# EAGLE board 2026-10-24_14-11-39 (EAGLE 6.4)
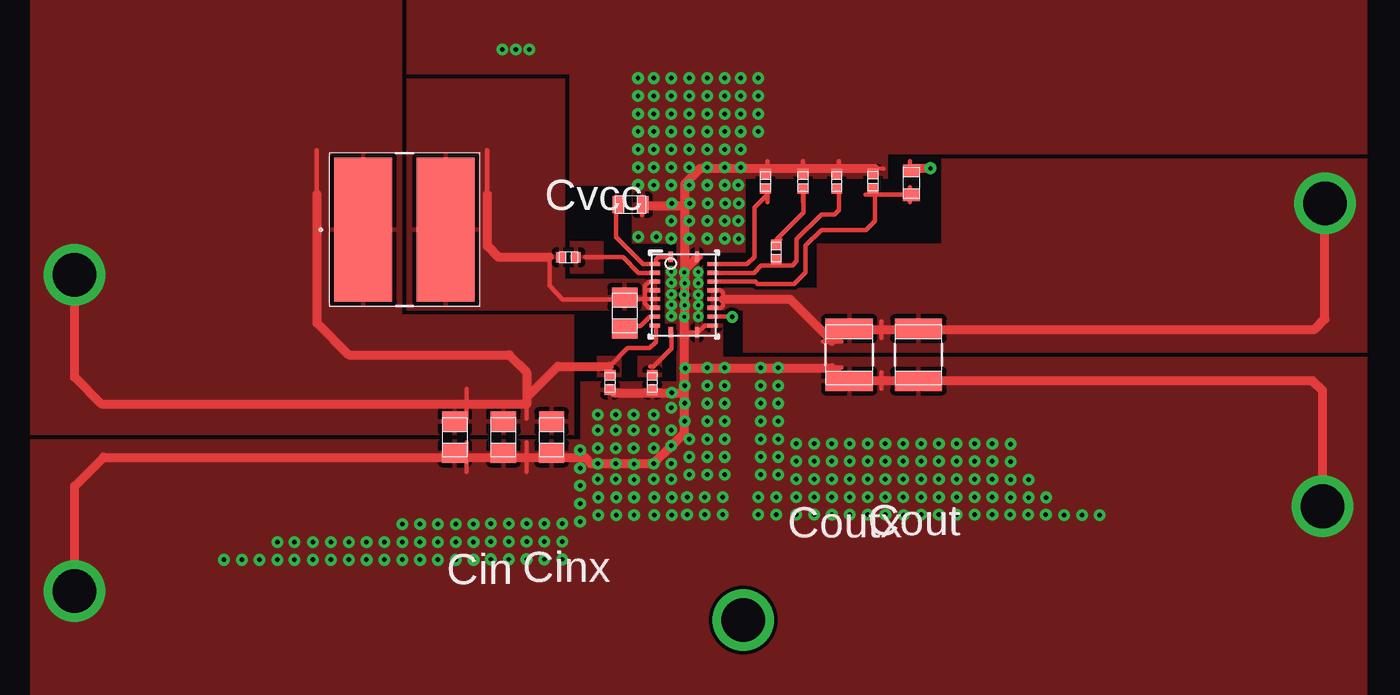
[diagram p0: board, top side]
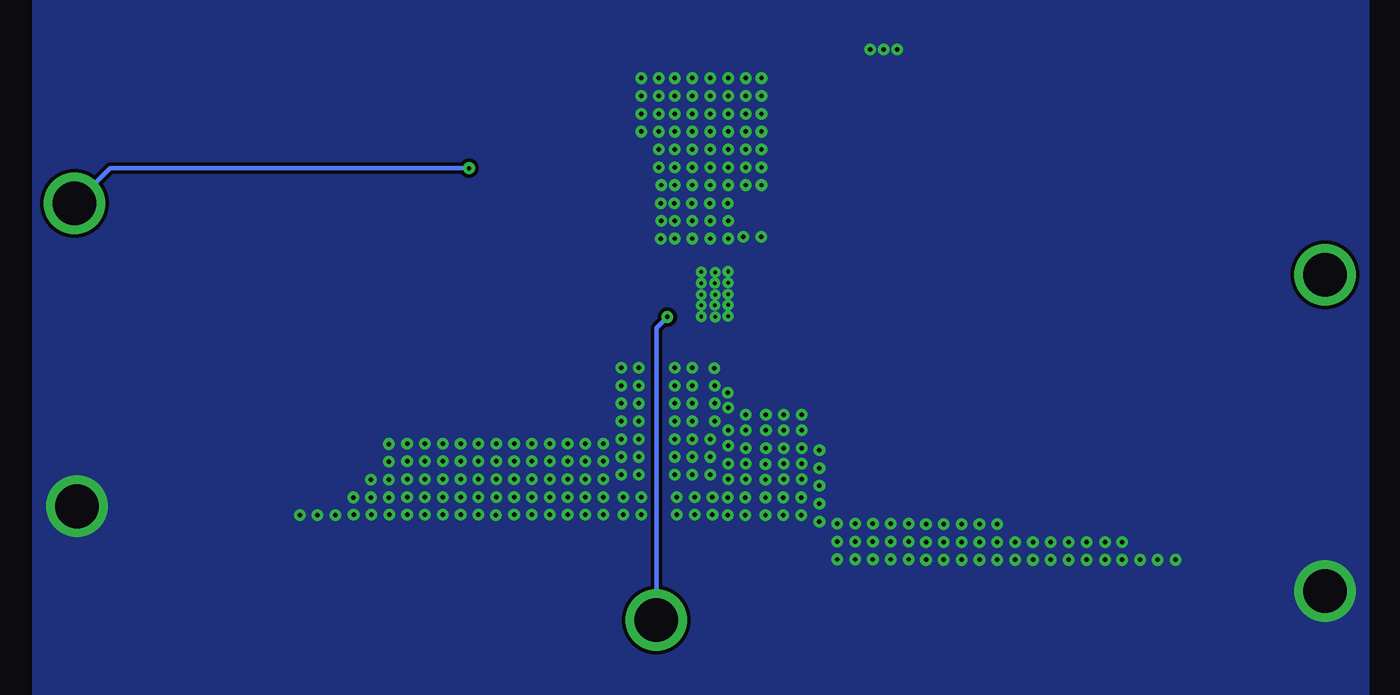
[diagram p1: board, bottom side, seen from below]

No outline drawn. Coordinates in mm, seen from the top.
Copper layers ((1*2)+(15*16)): TOP / INTERNAL1 / layer 15 / BOTTOM

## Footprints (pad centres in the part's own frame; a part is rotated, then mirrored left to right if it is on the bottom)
0805 = smd 1.118 x 1.448: 1 -0.902,0; 2 0.902,0
0402 = smd 0.559 x 0.61: 1 -0.419,0; 2 0.419,0
1210_280 = smd 1.118 x 2.692: 1 -1.499,0; 2 1.499,0
0603 = smd 0.66 x 0.965: 1 -0.699,0; 2 0.699,0
TP-1502 = drill 0.813 pad 1.651 round: 1 0,0
VLP8040 = smd 3.302 x 8.204: 1 -2.349,0; 2 2.349,0
RHL0020A = smd 0.24 x 0.6: 1 -0.75,2.15; 10 -0.75,-2.15; 11 0.75,-2.15; 20 0.75,2.15 | smd 0.6 x 0.24: 2 -1.65,1.75; 3 -1.65,1.25; 4 -1.65,0.75; 5 -1.65,0.25; 6 -1.65,-0.25; 7 -1.65,-0.75; 8 -1.65,-1.25; 9 -1.65,-1.75; 12 1.65,-1.75; 13 1.65,-1.25; 14 1.65,-0.75; 15 1.65,-0.25; 16 1.65,0.25; 17 1.65,0.75; 18 1.65,1.25; 19 1.65,1.75 | smd 0.3 x 0.3: 21 0,0

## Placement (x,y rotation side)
Cbst  [0805]  60.55,53.7 270 top
Ccomp  [0402]  70.71,61.19 90 top
Ccomp2  [0402]  72.64,61.19 90 top
Cin2  [0402]  59.72,49.73 270 top
Cin_1  [0805]  56.39,46.61 270 top
Cin_2  [0805]  53.64,46.61 270 top
Cin_3  [0805]  50.88,46.61 270 top
Cout_1  [1210_280]  73.36,51.31 270 top
Cout_2  [1210_280]  77.29,51.31 270 top
Css  [0402]  62.13,49.73 270 top
Cvcc_1  [0603]  60.88,59.87 0 top
Cvcc_2  [0603]  60.88,59.87 0 top
GND  [TP-1502]  29.18,37.85 270 top
GND1  [TP-1502]  100.28,42.65 270 top
L1  [VLP8040]  48.01,58.45 0 top
MODE  [TP-1502]  67.28,36.2 270 top
Rcomp  [0402]  69.19,57.18 90 top
Rfbb  [0402]  74.7,61.21 90 top
Rfbt  [0603]  76.89,61.11 270 top
Rlim  [0402]  68.58,61.19 90 top
Rt  [0402]  57.35,56.87 0 top
U1  [RHL0020A]  63.93,54.74 0 top
VIN  [TP-1502]  29.18,55.83 270 top
VOUT  [TP-1502]  100.38,59.89 270 top

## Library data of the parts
Cbst = ultra-librarian; RefDes: Cbst; Type: 08053C104KAT2A
Ccomp = ultra-librarian; RefDes: Ccomp; Type: GRM1555C1E751JA01D
Ccomp2 = ultra-librarian; RefDes: Ccomp2; Type: GRM1555C1E390JA01D
Cin2 = ultra-librarian; RefDes: Cin2; Type: GRM155R71A104KA01D
Cin_1-Cin_3 Cout_1 Cout_2 Cvcc_1 Cvcc_2 = ultra-librarian
Css = ultra-librarian; RefDes: Css; Type: GRM155R71C822KA01D
GND = ultra-librarian; RefDes: GND; Type: TP-1502
GND1 = ultra-librarian; RefDes: GND1; Type: TP-1502
L1 = ultra-librarian; RefDes: L1; Type: VLP8040T-1R0N
MODE = ultra-librarian; RefDes: MODE; Type: TP-1502
Rcomp = ultra-librarian; RefDes: Rcomp; Type: CRCW040226K7FKED
Rfbb = ultra-librarian; RefDes: Rfbb; Type: CRCW040269K8FKED
Rfbt = ultra-librarian; RefDes: Rfbt; Type: RC0603FR-07220KL
Rlim = ultra-librarian; RefDes: Rlim; Type: CRCW0402154KFKED
Rt = ultra-librarian; RefDes: Rt; Type: CRCW0402267KFKED
U1 = ultra-librarian; RefDes: U1; Type: TPS61088RHLR
VIN = ultra-librarian; RefDes: VIN; Type: TP-1502
VOUT = ultra-librarian; RefDes: VOUT; Type: TP-1502

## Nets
0: Ccomp2.2 Ccomp.2 Cin2.2 Cin_1.2 Cin_2.2 Cin_3.2 Cout_1.2 Cout_2.2 Css.2 Cvcc_1.2 Cvcc_2.2 GND1.1 GND.1 Rfbb.2 Rlim.2 U1.11 U1.12 U1.20 U1.21
2: Cin2.1 Cin_1.1 Cin_2.1 Cin_3.1 L1.1 U1.9 VIN.1
3: Ccomp.1 Rcomp.2
4: Cvcc_1.1 Cvcc_2.1 U1.1 U1.2
5: Ccomp2.1 Rcomp.1 U1.18
9: Cout_1.1 Cout_2.1 Rfbt.1 U1.14 U1.15 U1.16 VOUT.1
11: Rfbb.1 Rfbt.2 U1.17
12: Cbst.1 L1.2 Rt.1 U1.4 U1.5 U1.6 U1.7
14: Rlim.1 U1.19
17: Css.1 U1.10
18: Cbst.2 U1.8
19: Rt.2 U1.3
25: MODE.1 U1.13

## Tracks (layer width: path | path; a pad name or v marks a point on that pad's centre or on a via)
0  (via drill 0.2 pad 0.48, 0.25 pad 0.51, 2.49 pad 3.48)
  TOP 0.254: 65.61,52.98 65.13,52.98 64.72,52.58 63.98,52.58 63.96,52.58 | 74.27,61.94 75.31,61.94 | 72.76,61.52 72.76,62.36 | 70.73,61.52 70.73,62.36 | 68.69,61.52 68.69,62.36 | 71.86,50.58 72.9,50.58 | 61.56,59.28 61.56,60.33 | 54.97,44.63 54.97,46.3 | 75.18,49.38 75.18,50.32 | 51.54,44.63 51.54,46.3
  TOP 0.508: 63.98,59.82 63.98,60.98 63.98,61.06 64.87,61.95 68.71,61.95 70.74,61.95 | 63.98,59.82 63.98,58.95 63.98,56.16 | 63.98,56.16 v63.98,55.4 v63.98,54.13 63.98,53.49 v63.96,53.47 63.96,52.58 63.96,50.67 | 61.57,59.82 63.98,59.82 | 63.96,49.4 63.96,50.67 | 63.96,49.4 63.96,46.86 v63.22,46.13 v62.2,45.11 v60.05,45.11 v59.03,45.11 58.62,45.11 58.29,45.47 54.99,45.47 51.56,45.47 30.86,45.47 29.21,43.81 v29.21,37.85 | 59.69,49.4 59.94,49.15 62,49.15 63.73,49.15 63.96,49.4 | 63.96,50.67 64.03,50.57 v69.32,50.57 72.36,50.57 73.13,49.84 75.18,49.84 99.75,49.84 100.33,49.28 v100.33,42.67 | 63.98,56.16 64.72,56.9 | 59.69,49.4 | 63.96,49.4 | 70.74,61.95 72.77,61.95 74.8,61.95 | 70.74,61.95 | 74.8,61.95 | 61.57,59.82
  other vias: 63.22,54.76 63.96,56.01 64.74,54.74 63.22,53.52 63.22,54.15 63.22,56.06 37.72,39.62 39.75,39.62 41.73,39.62 67.06,59.94 87.63,42.16 86.61,42.16 85.6,42.16 84.58,43.18 83.57,43.18 82.55,45.21 82.55,44.2 82.55,43.18 82.55,46.23 40.77,39.62 40.77,40.64 41.73,40.64 42.8,39.62 42.8,40.64 43.81,39.62 43.81,40.64 44.83,39.62 44.83,40.64 45.85,39.62 45.85,40.64 55.12,68.71 76.45,42.16 64.01,50.55 69.19,43.21 58.01,44.86 63.22,48.29 73.38,46.25 63.96,54.74 48.9,40.64 48.9,39.62 48.9,41.66 60.07,42.16 60.07,43.18 47.88,41.66 47.88,39.62 47.88,40.64 46.86,40.64 46.86,39.62 61.09,43.18 61.09,42.16 49.91,41.66 49.91,39.62 49.91,40.64 50.93,40.64 50.93,39.62 50.93,41.66 62.23,42.16 62.23,43.18 64.74,54.13 64.74,53.49 64.74,55.4 63.22,55.42 64.74,56.03 68.3,50.57 66.27,50.57 65.25,50.57 68.3,49.56 65.25,49.56 66.27,49.56 66.27,47.52 63.22,47.02 63.98,47.52 65.25,47.52 60.05,47.9 59.03,47.9 68.17,43.21 66.14,43.21 58.01,45.87 64.11,43.21 63.25,43.18 65.13,43.21 69.32,49.56 64.11,42.19 63.25,42.16 69.19,42.19 65.13,42.19 66.14,42.19 68.17,42.19 61.06,47.02 59.03,47.02 60.05,47.02 62.2,47.02 79.48,45.24 74.4,45.24 72.36,45.24 73.38,45.24 78.46,45.24 75.41,45.24 76.43,45.24 77.44,45.24 70.33,45.24 69.32,47.52 68.3,47.52 71.35,45.24 71.35,44.22 68.3,46.51 69.32,46.51 70.33,44.22 77.44,44.22 76.43,44.22 75.41,44.22 78.46,44.22 73.38,44.22 72.36,44.22 74.4,44.22 79.48,44.22 60.05,46 59.03,46 58.01,43.84 61.06,46 55.98,41.68 54.97,41.68 53.95,41.68 57,41.68 51.94,41.66 52.93,41.68 65.25,46.51 64.24,46.51 66.27,46.51 66.27,44.48 63.22,44.22 64.24,44.48 65.25,44.48 52.93,39.65 51.94,39.62 57,39.65 53.95,39.65 54.97,39.65 55.98,39.65 61.09,44.2 58.01,41.81 59.03,44.22 60.05,44.22 62.2,44.22 79.48,42.19 74.4,42.19 72.36,42.19 73.38,42.19 78.46,42.19 75.41,42.19 77.44,42.19 70.33,42.19 69.32,44.48 68.3,44.48 71.35,42.19 71.35,43.21 68.3,45.49 69.32,45.49 70.33,43.21 77.44,43.21 76.43,43.21 75.41,43.21 78.46,43.21 73.38,43.21 72.36,43.21 74.4,43.21 79.48,43.21 58.01,42.82 55.98,40.67 54.97,40.67 53.95,40.67 57,40.67 51.94,40.64 52.93,40.67 65.25,45.49 64.24,45.49 63.22,45.11 66.27,45.49 83.54,42.19 80.49,42.19 81.51,42.19 82.52,42.19 84.56,42.19 65.25,57.94 63.22,57.94 64.24,57.94 66.27,57.94 65.25,58.95 63.22,58.95 64.24,58.95 66.27,58.95 66.29,59.94 63.25,59.94 64.26,59.94 65.28,59.94 66.27,60.99 63.22,60.99 64.24,60.99 65.25,60.99 67.03,60.99 61.32,62 67.16,62 65.25,62 64.24,62 63.22,62 66.27,62 62.2,63.02 66.27,63.02 63.22,63.02 64.24,63.02 65.25,63.02 67.16,63.02 68.17,64.03 67.16,64.03 65.25,64.03 64.24,64.03 63.22,64.03 66.27,64.03 62.2,64.03 62.2,65.05 66.27,65.05 63.22,65.05 64.24,65.05 65.25,65.05 67.16,65.05 68.17,65.05 68.17,66.07 67.16,66.07 65.25,66.07 64.24,66.07 63.22,66.07 66.27,66.07 62.2,66.07 68.17,67.08 67.16,67.08 65.25,67.08 64.24,67.08 63.22,67.08 66.27,67.08 62.2,67.08 61.32,60.99 62.2,62 62.2,60.99 71.35,46.25 68.3,48.54 69.32,48.54 70.33,46.25 77.44,46.25 76.43,46.25 75.41,46.25 78.46,46.25 72.36,46.25 74.4,46.25 79.48,46.25 62.2,47.9 61.06,47.9 65.25,48.54 66.27,48.54 81.51,46.25 80.49,46.25 81.51,43.21 80.49,43.21 81.51,44.22 80.49,44.22 80.49,45.24 81.51,45.24 61.32,67.08 61.32,66.07 61.32,65.05 61.32,64.03 61.32,63.02 63.25,49.15 59.05,42.16 59.05,43.18 53.59,68.71 38.73,39.62 54.36,68.71 63.98,49.56 63.98,48.54 62.2,46 61.09,45.09 83.57,44.2 62.36,58.04 61.34,58.04 67.06,57.91 67.03,58.95
  pour TOP: 58.04,49.78 63.5,49.78 63.5,53.09 62.87,53.09 62.87,56.39 63.5,56.39 63.5,57.66 60.96,57.66 60.96,60.96 57.4,60.96 57.4,67.31 48.13,67.31 48.13,82.55 102.87,82.55 102.87,62.74 75.56,62.74 75.56,61.34 67.44,61.34 67.44,57.15 65.02,57.15 65.02,53.09 66.17,53.09 66.17,51.18 102.87,51.18 102.87,26.67 26.67,26.67 26.67,46.48 58.04,46.48
  pour BOTTOM: 26.67,26.67 26.67,82.55 102.87,82.55 102.87,26.67
2  (via drill 2.49 pad 3.48)
  TOP 0.254: 59.69,50.65 60.71,51.69 61.98,51.69 62.33,52.05 62.33,52.98 | 54.97,47.68 54.97,49.35 | 43,57.94 43,62.97 | 51.54,47.68 51.54,49.35
  TOP 0.508: 54.99,48.9 54.99,50.29 53.98,51.31 44.83,51.31 43.03,53.11 43.03,60.45 | 54.99,48.9 54.99,48.51 51.56,48.51 30.73,48.51 29.21,50.04 v29.21,55.88 | 59.69,50.65 56.74,50.65 54.99,48.9
  pour TOP: 58.98,50.04 58.98,51.23 60.38,51.23 60.38,50.04
  pour TOP (rank 4): 47.88,82.55 47.88,53.59 57.66,53.59 57.66,46.74 26.67,46.74 26.67,82.55
3
  TOP 0.254: 69.44,57.89 69.22,57.89 70.74,59.41 70.74,60.45 | 70.73,60.02 70.73,60.86
4
  TOP 0.254: 63.22,56.9 62.48,56.9 62.33,56.74 62.33,56.49 61.59,56.49 60.07,58.01 60.07,59.82 | 60.06,59.28 60.06,60.33
5
  TOP 0.254: 65.61,55.98 67.92,55.98 68.33,56.39 69.22,56.39 70.1,56.39 70.36,56.64 70.36,57.91 71.75,59.31 72.52,59.31 72.77,59.56 72.77,60.45 | 72.76,60.02 72.76,60.86
9  (via drill 0.25 pad 0.51, 2.49 pad 3.48)
  TOP 0.254: 65.61,54.99 66.02,54.99 66.17,54.86 66.17,54.48 | 65.61,53.98 66.04,53.98 66.17,54.1 66.17,54.48 | 65.61,54.48 66.17,54.48 | 76.82,61.52 76.82,62.36 | 71.86,52.08 72.9,52.08 | 75.18,52.27 75.18,53.21
  TOP 0.508: v100.46,59.94 100.46,53.34 99.87,52.76 75.18,52.76 73.05,52.76 72.36,52.09 69.98,54.48 66.17,54.48 | 76.83,61.95 v77.98,61.95
  BOTTOM 0.254: v100.46,59.94 98.42,61.95 v77.98,61.95
  pour TOP (rank 6): 65.28,53.85 65.28,55.12 71.5,55.12 71.5,57.66 78.61,57.66 78.61,62.48 102.87,62.48 102.87,51.44 67.31,51.44 67.31,53.85
11
  TOP 0.254: 65.61,55.5 68,55.5 68.12,55.35 70.21,55.35 70.87,56.01 70.87,57.53 71.75,58.42 74.3,58.42 74.8,58.93 74.8,60.45 | 74.8,60.45 76.83,60.45 | 74.8,60.45 | 76.82,60.02 76.82,60.86 | 74.27,60.44 75.31,60.44
12
  TOP 0.254: 62.33,55.5 61.98,55.5 61.72,55.24 61.72,54.99 | 62.33,53.98 61.95,53.98 61.72,54.23 61.72,54.48 | 61.72,54.48 62.33,54.48 | 61.72,54.99 62.33,54.99 | 61.72,54.99 | 61.72,54.48 60.6,54.48 60.58,54.46 57.02,54.46 56.26,55.24 56.26,56.9 | 61.72,54.48 61.72,54.99 | 52.7,57.94 52.7,62.97
  TOP 0.508: 52.73,60.45 52.73,57.51 53.34,56.9 56.26,56.9
  pour TOP (rank 5): 48.13,53.85 48.13,67.06 57.15,67.06 57.15,55.63 62.61,55.63 62.61,53.85
14
  TOP 0.254: 65.61,56.49 67.54,56.49 67.94,56.9 67.94,59.69 68.71,60.45 | 68.69,60.02 68.69,60.86
17
  TOP 0.254: 63.22,52.58 63.22,51.66 62.2,50.65 62,50.65
  pour TOP (rank 2): 61.29,50.04 61.29,51.23 62.69,51.23 62.69,50.04
18
  TOP 0.254: 60.58,52.96 61.47,52.96 62,53.49 62.33,53.49
19
  TOP 0.254: 62.33,55.98 61.34,55.98 60.45,56.9 58.29,56.9
  pour TOP (rank 3): 57.45,55.96 57.45,57.78 59.36,57.78 59.36,55.96
25  (via drill 0.25 pad 0.51, 2.49 pad 3.48)
  TOP 0.254: v66.67,53.47 66.62,53.49 65.61,53.49
  BOTTOM 0.254: v67.31,36.2 67.31,52.83 v66.67,53.47

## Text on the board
ASSYNOTES: Design Rules: Min Clearance: 10mil | Min Track Width: 10mil | Cvcc | Coutx | Cout | Cin | Cinx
